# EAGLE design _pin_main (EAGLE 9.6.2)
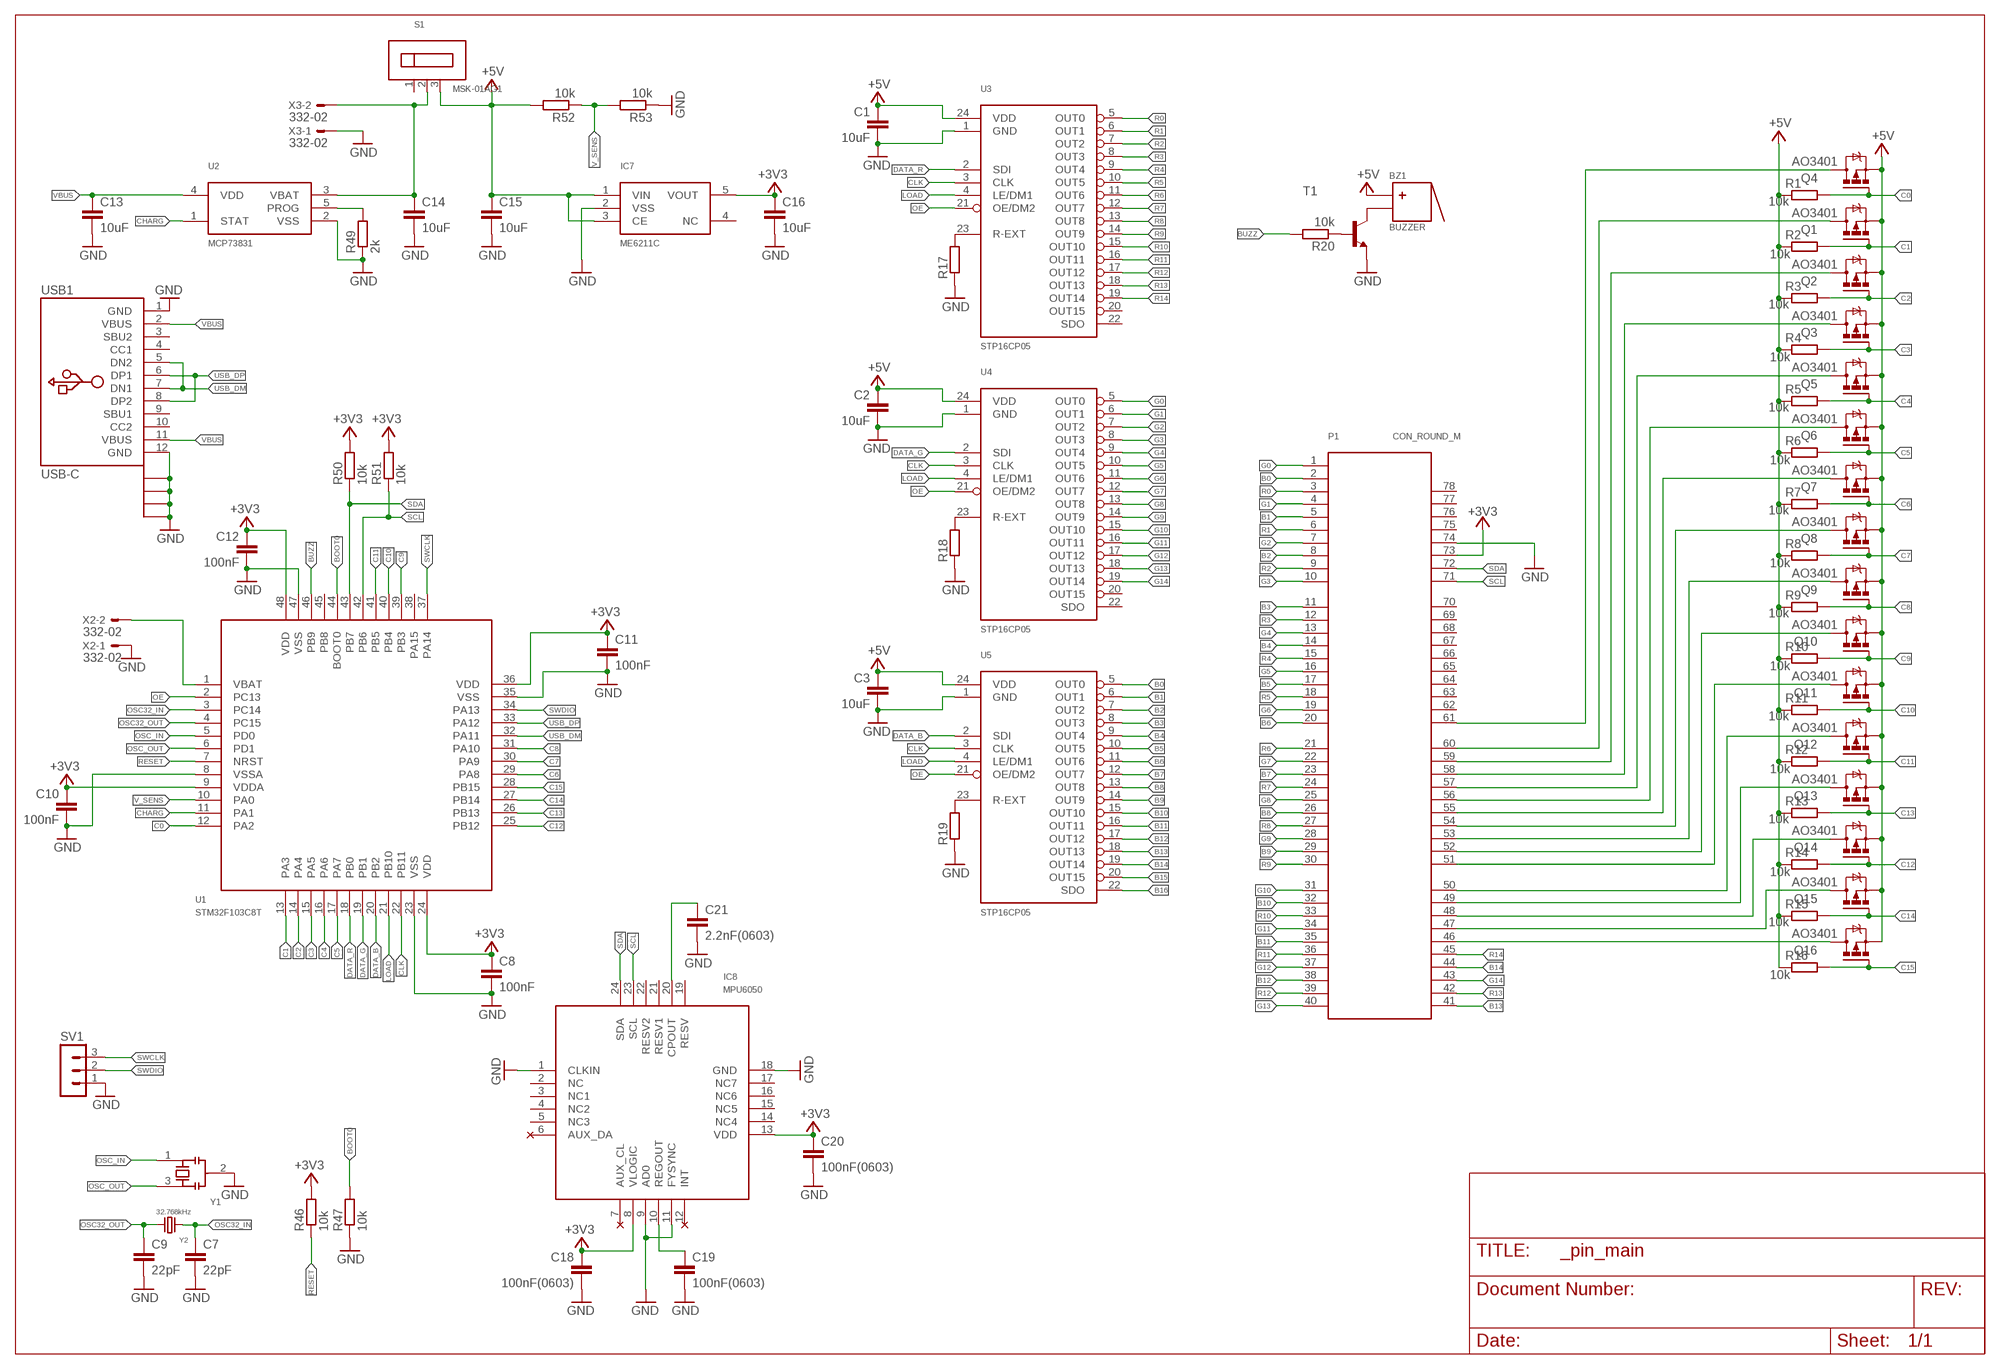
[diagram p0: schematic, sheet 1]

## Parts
BZ1  BUZZER  [HCT9032B]
C1  10uF  C-EUC0402K  [C0402K]
C2  10uF  C-EUC0402K  [C0402K]
C3  10uF  C-EUC0402K  [C0402K]
C7  22pF  C-EUC0402K  [C0402K]
C8  100nF  C-EUC0402K  [C0402K]
C9  22pF  C-EUC0402K  [C0402K]
C10  100nF  C-EUC0402K  [C0402K]
C11  100nF  C-EUC0402K  [C0402K]
C12  100nF  C-EUC0402K  [C0402K]
C13  10uF  C-EUC0805  [C0805]
C14  10uF  C-EUC0805  [C0805]
C15  10uF  C-EUC0805  [C0805]
C16  10uF  C-EUC0805  [C0805]
C18  100nF(0603)  C-EUC0402K  [C0402K]
C19  100nF(0603)  C-EUC0402K  [C0402K]
C20  100nF(0603)  C-EUC0402K  [C0402K]
C21  2.2nF(0603)  C-EUC0402K  [C0402K]
IC7  ME6211C  [SOT23-5]
IC8  MPU6050  [QFN24-4X4]
P1  CON_ROUND_M  [CON_61_M]
Q1  AO3401  IRLML5203  [MICRO3]
Q2  AO3401  IRLML5203  [MICRO3]
Q3  AO3401  IRLML5203  [MICRO3]
Q4  AO3401  IRLML5203  [MICRO3]
Q5  AO3401  IRLML5203  [MICRO3]
Q6  AO3401  IRLML5203  [MICRO3]
Q7  AO3401  IRLML5203  [MICRO3]
Q8  AO3401  IRLML5203  [MICRO3]
Q9  AO3401  IRLML5203  [MICRO3]
Q10  AO3401  IRLML5203  [MICRO3]
Q11  AO3401  IRLML5203  [MICRO3]
Q12  AO3401  IRLML5203  [MICRO3]
Q13  AO3401  IRLML5203  [MICRO3]
Q14  AO3401  IRLML5203  [MICRO3]
Q15  AO3401  IRLML5203  [MICRO3]
Q16  AO3401  IRLML5203  [MICRO3]
R1  10k  R-EU_R0402  [R0402]
R2  10k  R-EU_R0402  [R0402]
R3  10k  R-EU_R0402  [R0402]
R4  10k  R-EU_R0402  [R0402]
R5  10k  R-EU_R0402  [R0402]
R6  10k  R-EU_R0402  [R0402]
R7  10k  R-EU_R0402  [R0402]
R8  10k  R-EU_R0402  [R0402]
R9  10k  R-EU_R0402  [R0402]
R10  10k  R-EU_R0402  [R0402]
R11  10k  R-EU_R0402  [R0402]
R12  10k  R-EU_R0402  [R0402]
R13  10k  R-EU_R0402  [R0402]
R14  10k  R-EU_R0402  [R0402]
R15  10k  R-EU_R0402  [R0402]
R16  10k  R-EU_R0402  [R0402]
R17  R-EU_R0603  [R0603]
R18  R-EU_R0603  [R0603]
R19  R-EU_R0603  [R0603]
R20  10k  R-EU_R0402  [R0402]
R46  10k  R-EU_R0402  [R0402]
R47  10k  R-EU_R0402  [R0402]
R49  2k  R-EU_R0603  [R0603]
R50  10k  R-EU_R0402  [R0402]
R51  10k  R-EU_R0402  [R0402]
R52  10k  R-EU_R0402  [R0402]
R53  10k  R-EU_R0402  [R0402]
S1  MSK-01AG1  [MSK-01AG1]
SV1  MA03-1  [MA03-1]
T1  BC849-NPN-SOT23-BEC  [SOT23-BEC]
U1  STM32F103C8T  [LQFP48-7X7]
U2  MCP73831  [SOT23-5]
U3  STP16CP05  [TSSOP24]
U4  STP16CP05  [TSSOP24]
U5  STP16CP05  [TSSOP24]
USB1  USB-C  [USB-C-A40-00119]
X2  332-02  [332-02]
X3  332-02  [332-02]
Y1  XTAL_CSTCE  [CSTCE]
Y2  32.768kHz  WE-XTAL_WATCH_830002997B_2X6  [WE-XTAL_WATCH-2X6]

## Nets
+3V3: C8.1 C10.1 C11.1 C12.1 C16.1 C18.1 C20.1 IC7.5(VOUT) IC8.8(VLOGIC) IC8.13(VDD) P1.73 R46.2 R50.2 R51.2 U1.9(VDDA) U1.24(VDD) U1.36(VDD) U1.48(VDD)
+5V: BZ1.1 C1.1 C2.1 C3.1 C15.1 IC7.1(VIN) IC7.3(CE) Q1.2(S) Q2.2(S) Q3.2(S) Q4.2(S) Q5.2(S) Q6.2(S) Q7.2(S) Q8.2(S) Q9.2(S) Q10.2(S) Q11.2(S) Q12.2(S) Q13.2(S) Q14.2(S) Q15.2(S) Q16.2(S) R1.1 R2.1 R3.1 R4.1 R5.1 R6.1 R7.1 R8.1 R9.1 R10.1 R11.1 R12.1 R13.1 R14.1 R15.1 R16.1 R52.2 S1.3 U3.24(VDD) U4.24(VDD) U5.24(VDD)
B0: P1.2 U5.5(OUT0)
B1: P1.5 U5.6(OUT1)
B2: P1.8 U5.7(OUT2)
B3: P1.11 U5.8(OUT3)
B4: P1.14 U5.9(OUT4)
B5: P1.17 U5.10(OUT5)
B6: P1.20 U5.11(OUT6)
B7: P1.23 U5.12(OUT7)
B8: P1.26 U5.13(OUT8)
B9: P1.29 U5.14(OUT9)
B10: P1.32 U5.15(OUT10)
B11: P1.35 U5.16(OUT11)
B12: P1.38 U5.17(OUT12)
B13: P1.41 U5.18(OUT13)
B14: P1.44 U5.19(OUT14)
B15: U5.20(OUT15)
B16: U5.22(SDO)
BOOT0: R47.2 U1.44(BOOT0)
BUZZ: R20.2 U1.46(PB9)
C0: Q4.1(G) R1.2 U1.12(PA2)
C1: Q1.1(G) R2.2 U1.13(PA3)
C2: Q2.1(G) R3.2 U1.14(PA4)
C3: Q3.1(G) R4.2 U1.15(PA5)
C4: Q5.1(G) R5.2 U1.16(PA6)
C5: Q6.1(G) R6.2 U1.17(PA7)
C6: Q7.1(G) R7.2 U1.29(PA8)
C7: Q8.1(G) R8.2 U1.30(PA9)
C8: Q9.1(G) R9.2 U1.31(PA10)
C9: Q10.1(G) R10.2 U1.39(PB3)
C10: Q11.1(G) R11.2 U1.40(PB4)
C11: Q12.1(G) R12.2 U1.41(PB5)
C12: Q14.1(G) R14.2 U1.25(PB12)
C13: Q13.1(G) R13.2 U1.26(PB13)
C14: Q15.1(G) R15.2 U1.27(PB14)
C15: Q16.1(G) R16.2 U1.28(PB15)
CHARG: U1.11(PA1) U2.1(STAT)
CLK: U1.22(PB11) U3.3(CLK) U4.3(CLK) U5.3(CLK)
DATA_B: U1.20(PB2) U5.2(SDI)
DATA_G: U1.19(PB1) U4.2(SDI)
DATA_R: U1.18(PB0) U3.2(SDI)
G0: P1.1 U4.5(OUT0)
G1: P1.4 U4.6(OUT1)
G2: P1.7 U4.7(OUT2)
G3: P1.10 U4.8(OUT3)
G4: P1.13 U4.9(OUT4)
G5: P1.16 U4.10(OUT5)
G6: P1.19 U4.11(OUT6)
G7: P1.22 U4.12(OUT7)
G8: P1.25 U4.13(OUT8)
G9: P1.28 U4.14(OUT9)
G10: P1.31 U4.15(OUT10)
G11: P1.34 U4.16(OUT11)
G12: P1.37 U4.17(OUT12)
G13: P1.40 U4.18(OUT13)
G14: P1.43 U4.19(OUT14)
GND: C1.2 C2.2 C3.2 C7.2 C8.2 C9.2 C10.2 C11.2 C12.2 C13.2 C14.2 C15.2 C16.2 C18.2 C19.2 C20.2 C21.2 IC7.2(VSS) IC8.1(CLKIN) IC8.9(AD0) IC8.11(FYSYNC) IC8.18(GND) P1.74 R17.1 R18.1 R19.1 R47.1 R49.1 R53.1 SV1.1 T1.E U1.8(VSSA) U1.23(VSS) U1.35(VSS) U1.47(VSS) U2.2(VSS) U3.1(GND) U4.1(GND) U5.1(GND) USB1.1(GND) USB1.12(GND) USB1.A(EXT) USB1.B(EXT1) USB1.C(EXT2) USB1.D(EXT3) X2.1 X3.1 Y1.2(GND)
LOAD: U1.21(PB10) U3.4(LE/DM1) U4.4(LE/DM1) U5.4(LE/DM1)
N$1: R17.2 U3.23(R-EXT)
N$2: R18.2 U4.23(R-EXT)
N$3: R19.2 U5.23(R-EXT)
N$4: BZ1.2 T1.C
N$5: R20.1 T1.B
N$49: U1.1(VBAT) X2.2
N$50: P1.46 Q16.3(D)
N$51: R49.2 U2.5(PROG)
N$52: C19.1 IC8.10(REGOUT)
N$53: C21.1 IC8.20(CPOUT)
N$54: P1.47 Q15.3(D)
N$55: C14.1 S1.2 U2.3(VBAT) X3.2
N$56: P1.48 Q14.3(D)
N$57: P1.49 Q13.3(D)
N$58: P1.50 Q12.3(D)
N$59: P1.51 Q11.3(D)
N$60: P1.52 Q10.3(D)
N$61: P1.53 Q9.3(D)
N$62: P1.54 Q8.3(D)
N$63: P1.55 Q7.3(D)
N$64: P1.56 Q6.3(D)
N$65: P1.57 Q5.3(D)
N$66: P1.58 Q3.3(D)
N$67: P1.59 Q2.3(D)
N$68: P1.60 Q1.3(D)
N$69: P1.61 Q4.3(D)
OE: U1.2(PC13) U3.21(OE/DM2) U4.21(OE/DM2) U5.21(OE/DM2)
OSC32_IN: C7.1 U1.3(PC14) Y2.1
OSC32_OUT: C9.1 U1.4(PC15) Y2.2
OSC_IN: U1.5(PD0) Y1.1(XI)
OSC_OUT: U1.6(PD1) Y1.3(XO)
R0: P1.3 U3.5(OUT0)
R1: P1.6 U3.6(OUT1)
R2: P1.9 U3.7(OUT2)
R3: P1.12 U3.8(OUT3)
R4: P1.15 U3.9(OUT4)
R5: P1.18 U3.10(OUT5)
R6: P1.21 U3.11(OUT6)
R7: P1.24 U3.12(OUT7)
R8: P1.27 U3.13(OUT8)
R9: P1.30 U3.14(OUT9)
R10: P1.33 U3.15(OUT10)
R11: P1.36 U3.16(OUT11)
R12: P1.39 U3.17(OUT12)
R13: P1.42 U3.18(OUT13)
R14: P1.45 U3.19(OUT14)
RESET: R46.1 U1.7(NRST)
SCL: IC8.23(SCL) P1.71 R51.1 U1.42(PB6)
SDA: IC8.24(SDA) P1.72 R50.1 U1.43(PB7)
SWCLK: SV1.3 U1.37(PA14)
SWDIO: SV1.2 U1.34(PA13)
USB_DM: U1.32(PA11) USB1.5(DN2) USB1.7(DN1)
USB_DP: U1.33(PA12) USB1.6(DP1) USB1.8(DP2)
V_SENS: R52.1 R53.2 U1.10(PA0)
VBUS: C13.1 U2.4(VDD) USB1.2(VBUS) USB1.11(VBUS)
Unconnected: IC7.4(NC) IC8.2(NC) IC8.3(NC1) IC8.4(NC2) IC8.5(NC3) IC8.6(AUX_DA) IC8.7(AUX_CL) IC8.12(INT) IC8.14(NC4) IC8.15(NC5) IC8.16(NC6) IC8.17(NC7) IC8.19(RESV) IC8.21(RESV1) IC8.22(RESV2) P1.62 P1.63 P1.64 P1.65 P1.66 P1.67 P1.68 P1.69 P1.70 P1.75 P1.76 P1.77 P1.78 S1.1 U1.38(PA15) U1.45(PB8) U3.20(OUT15) U3.22(SDO) U4.20(OUT15) U4.22(SDO) USB1.3(SBU2) USB1.4(CC1) USB1.9(SBU1) USB1.10(CC2)

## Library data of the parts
BZ1 = GUIDO_PCB_LIB:BUZZER
C1-C3 C7-C16 C18-C21 = my_rcl:C-EU: CAPACITOR, European symbol; SPICEPREFIX: C
IC7 = GUIDO_PCB_LIB:ME6211C
IC8 = controller_KRAI:MPU6050
P1 = GUIDO_PCB_LIB:CON_ROUND_M
Q1-Q16 = transistor-power:IRLML5203: HEXFET P-Channel Power MOSFET
R1-R20 R46 R47 R49-R53 = my_rcl:R-EU_: RESISTOR, European symbol; SPICEPREFIX: R
S1 = GUIDO_PCB_LIB:MSK-01AG1
SV1 = my_con-lstb:MA03-1: PIN HEADER; OC_FARNELL: unknown; OC_NEWARK: unknown
T1 = transistor-neu-to92:*-NPN-: NPN Transistror
U1 = GUIDO_PCB_LIB:STM32F103C8T
U2 = GUIDO_PCB_LIB:MCP73831
U3-U5 = GUIDO_PCB_LIB:STP16CP05
USB1 = GUIDO_PCB_LIB:USB-C
X2 X3 = con-garry:332-02: 2 Pin - 2mm Dual Row
Y1 = GUIDO_PCB_LIB:XTAL_CSTCE
Y2 = my_Wurth_Quartz Crystals & Oscillators_WE-XTAL:WE-XTAL_WATCH: WE-XTAL Watch Crystals; C-LOAD: 12.5pF; DATASHEET-URL: https://www.we-online.com/catalog/datasheet/830002997B.pdf; MOUNT: THT; PART-NUMBER: 830002997B; TOLERANCE: ±20ppm

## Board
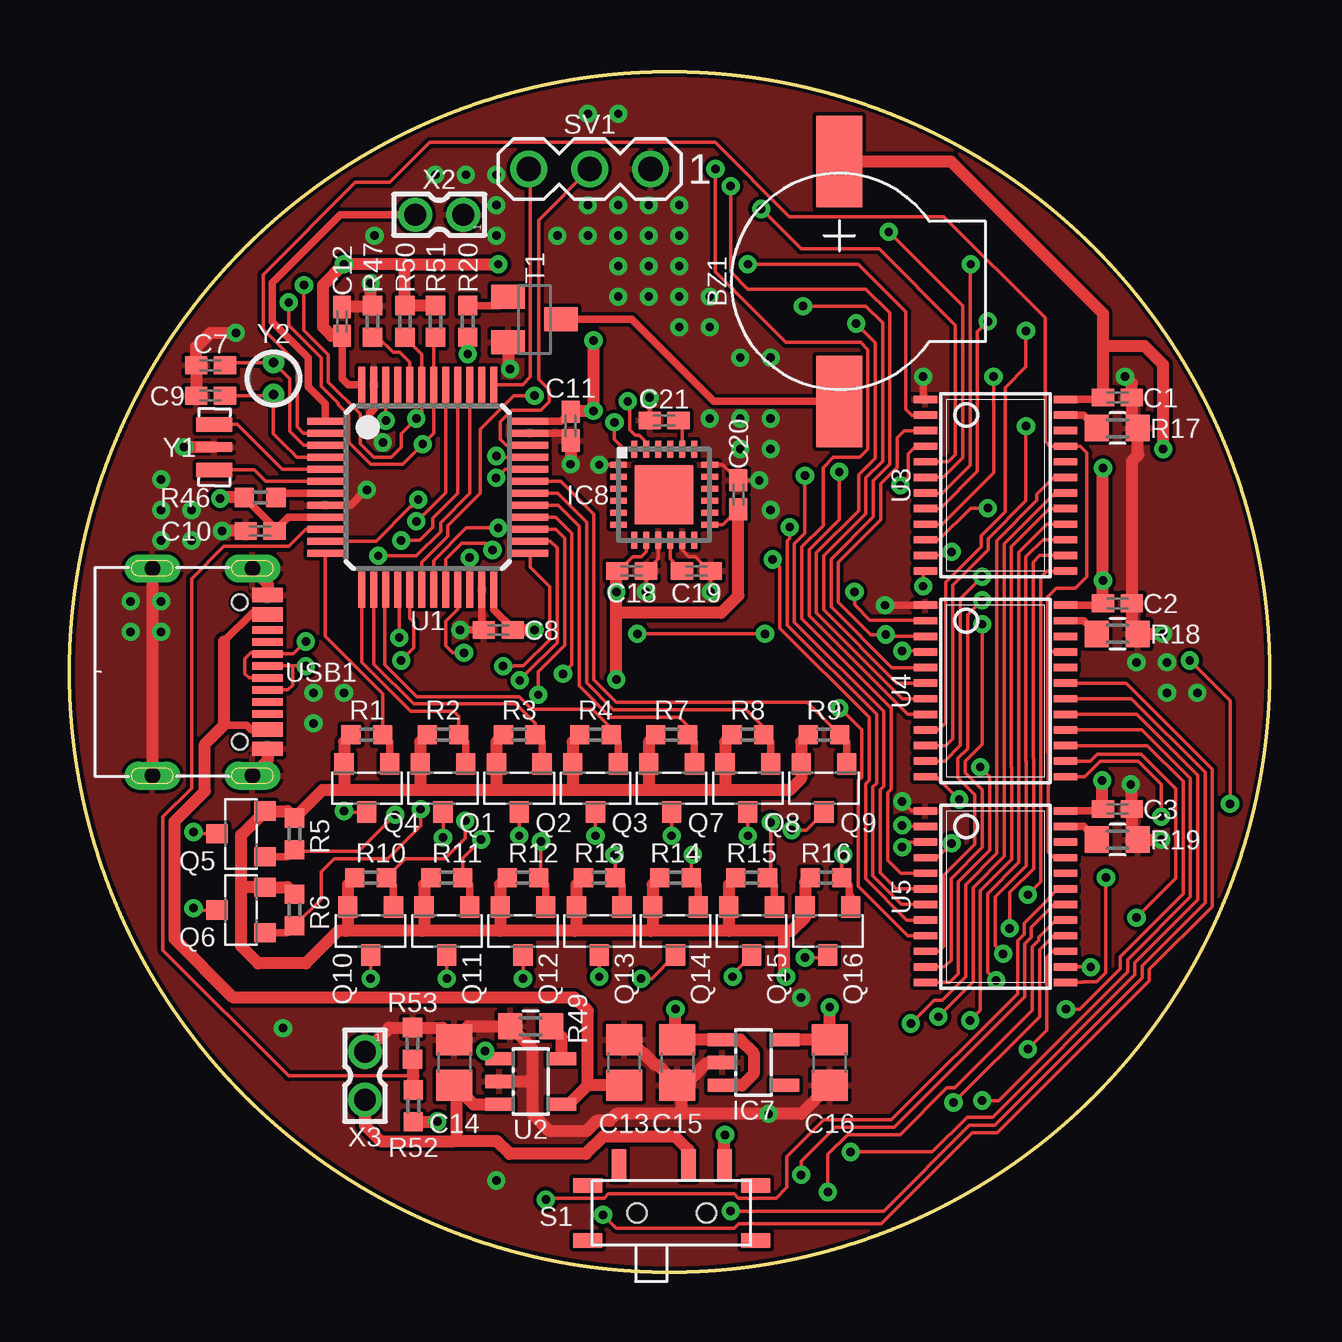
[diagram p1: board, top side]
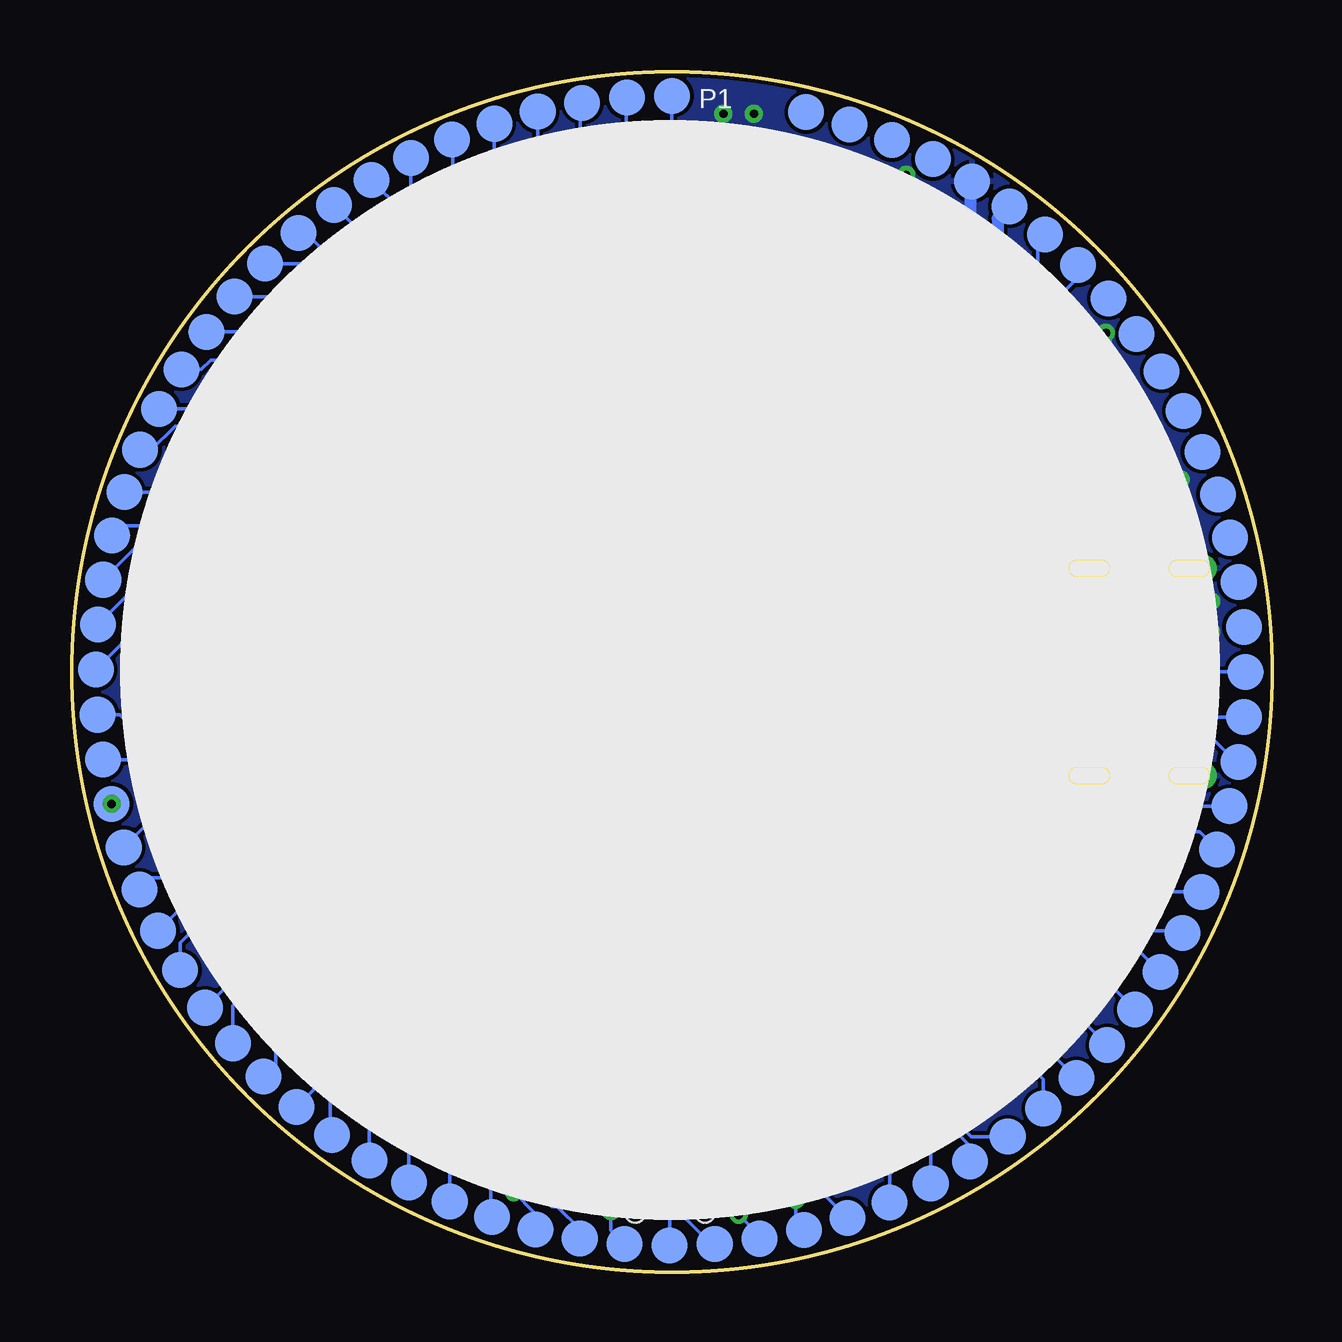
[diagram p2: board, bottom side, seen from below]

Size 50 x 50 mm. Coordinates in mm from the lower left corner, seen from the top.
Outline: circle at 25,25 radius 25
Copper layers (1*16): Top 0.035mm / dielectric 0.8mm / Bottom 0.035mm
Design rules "default *": minimum track width 6mil, minimum drill 0.35mm, track to track 6mil, track to pad 6mil, pad to pad 6mil, via to via 6mil, smd to smd 6mil, copper to edge 6mil, drill to drill 6mil, minimum pad ring 10mil, minimum via ring 8mil, stop-mask expansion 4mil, vias tented up to drill 0.35mm, thermal gap 6mil

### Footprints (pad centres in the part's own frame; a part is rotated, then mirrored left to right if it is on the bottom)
HCT9032B = smd 1.93 x 3.81: 1 0,5; 2 0,-5
C0402K = smd 0.925 x 0.74: 1 -0.6,0; 2 0.6,0
C0805 = smd 1.3 x 1.5: 1 -0.95,0; 2 0.95,0
SOT23-5 = smd 0.55 x 1.2: 1 -0.95,-1.3; 2 0,-1.3; 3 0.95,-1.3; 4 0.95,1.3; 5 -0.95,1.3
QFN24-4X4 = smd 0.7 x 0.25: 1 -1.9,1.25; 2 -1.9,0.75; 3 -1.9,0.25; 4 -1.9,-0.25; 5 -1.9,-0.75; 6 -1.9,-1.25; 13 1.9,-1.25; 14 1.9,-0.75; 15 1.9,-0.25; 16 1.9,0.25; 17 1.9,0.75; 18 1.9,1.25 | smd 0.25 x 0.7: 7 -1.25,-1.9; 8 -0.75,-1.9; 9 -0.25,-1.9; 10 0.25,-1.9; 11 0.75,-1.9; 12 1.25,-1.9; 19 1.25,1.9; 20 0.75,1.9; 21 0.25,1.9; 22 -0.25,1.9; 23 -0.75,1.9; 24 -1.25,1.9 | smd 2.45 x 2.45: EXP 0,0
CON_61_M = smd 1.5 x 1.5 bottom: 1 -24,0; 2 -23.93,1.879; 3 -23.713,3.747; 4 -23.35,5.593; 5 -22.843,7.404; 6 -22.195,9.17; 7 -21.412,10.879; 8 -20.496,12.522; 9 -19.454,14.088; 10 -18.293,15.567; 11 -17.019,16.95; 12 -15.641,18.23; 13 -14.166,19.397; 14 -12.605,20.445; 15 -10.966,21.367; 16 -9.259,22.158; 17 -7.496,22.813; 18 -5.687,23.327; 19 -3.843,23.698; 20 -1.976,23.922; 21 -0.097,24; 22 1.782,23.93; 23 3.65,23.713; 24 5.495,23.35; 25 7.307,22.843; 26 9.072,22.195; 27 10.782,21.412; 28 12.425,20.496; 29 13.99,19.454; 30 15.47,18.293; 31 16.853,17.019; 32 18.133,15.641; 33 19.3,14.166; 34 20.348,12.605; 35 21.27,10.966; 36 22.061,9.259; 37 22.716,7.496; 38 23.23,5.687; 39 23.6,3.844; 40 23.825,1.976; 41 23.903,0.097; 42 23.833,-1.782; 43 23.616,-3.65; 44 23.252,-5.495; 45 22.746,-7.306; 46 22.098,-9.072; 47 21.314,-10.782; 48 20.399,-12.424; 49 19.357,-13.99; 50 18.196,-15.47; 51 16.922,-16.853; 52 15.544,-18.133; 53 14.069,-19.3; 54 12.507,-20.348; 55 10.868,-21.27; 56 9.162,-22.061; 57 7.399,-22.715; 58 5.59,-23.23; 59 3.746,-23.6; 60 1.879,-23.825; 61 0,-23.903; 62 -1.879,-23.833; 63 -3.747,-23.615; 64 -5.593,-23.252; 65 -7.404,-22.746; 66 -9.169,-22.098; 67 -10.879,-21.314; 68 -12.522,-20.399; 69 -14.088,-19.357; 70 -15.567,-18.196; 71 -16.95,-16.922; 72 -18.23,-15.544; 73 -19.397,-14.069; 74 -20.445,-12.507; 75 -21.367,-10.868; 76 -22.158,-9.162; 77 -22.813,-7.399; 78 -23.327,-5.59
MICRO3 = smd 0.8 x 0.9: 1 -0.95,-1; 2 0.95,-1; 3 0,1
R0402 = smd 0.8 x 0.8: 1 -0.659,0; 2 0.659,0
R0603 = smd 1 x 1.1: 1 -0.85,0; 2 0.85,0
MSK-01AG1 = smd 1.3 x 0.6: 1 2,2.2; 2 2,-0.7; 3 2,-2.2 | smd 0.6 x 1.2: 4 1.15,3.5; 5 -1.15,3.5; 6 -1.15,-3.5; 7 1.15,-3.5 | hole 0.8: 0,1.45; 0,-1.45
MA03-1 = drill 1.016: 1 -2.54,0; 2 0,0; 3 2.54,0
SOT23-BEC = smd 1 x 1.4: B -0.95,-1.1; C 0,1.1; E 0.95,-1.1
LQFP48-7X7 = smd 1.5 x 0.3: 1 -4.268,2.75; 2 -4.268,2.25; 3 -4.268,1.75; 4 -4.268,1.25; 5 -4.268,0.75; 6 -4.268,0.25; 7 -4.268,-0.25; 8 -4.268,-0.75; 9 -4.268,-1.25; 10 -4.268,-1.75; 11 -4.268,-2.25; 12 -4.268,-2.75; 25 4.268,-2.75; 26 4.268,-2.25; 27 4.268,-1.75; 28 4.268,-1.25; 29 4.268,-0.75; 30 4.268,-0.25; 31 4.268,0.25; 32 4.268,0.75; 33 4.268,1.25; 34 4.268,1.75; 35 4.268,2.25; 36 4.268,2.75 | smd 0.3 x 1.5: 13 -2.75,-4.268; 14 -2.25,-4.268; 15 -1.75,-4.268; 16 -1.25,-4.268; 17 -0.75,-4.268; 18 -0.25,-4.268; 19 0.25,-4.268; 20 0.75,-4.268; 21 1.25,-4.268; 22 1.75,-4.268; 23 2.25,-4.268; 24 2.75,-4.268; 37 2.75,4.268; 38 2.25,4.268; 39 1.75,4.268; 40 1.25,4.268; 41 0.75,4.268; 42 0.25,4.268; 43 -0.25,4.268; 44 -0.75,4.268; 45 -1.25,4.268; 46 -1.75,4.268; 47 -2.25,4.268; 48 -2.75,4.268
TSSOP24 = smd 0.305 x 0.991: 1 -3.575,-2.918; 2 -2.925,-2.918; 3 -2.275,-2.918; 4 -1.625,-2.918; 5 -0.975,-2.918; 6 -0.325,-2.918; 7 0.325,-2.918; 8 0.975,-2.918; 9 1.625,-2.918; 10 2.275,-2.918; 11 2.925,-2.918; 12 3.575,-2.918; 13 3.575,2.918; 14 2.925,2.918; 15 2.275,2.918; 16 1.625,2.918; 17 0.975,2.918; 18 0.325,2.918; 19 -0.325,2.918; 20 -0.975,2.918; 21 -1.625,2.918; 22 -2.275,2.918; 23 -2.925,2.918; 24 -3.575,2.918
USB-C-A40-00119 = smd 0.6 x 1.27: 1 -3.2,7.2; 2 -2.4,7.2; 11 2.4,7.2; 12 3.2,7.2 | smd 0.3 x 1.27: 3 -1.75,7.2; 4 -1.25,7.2; 5 -0.75,7.2; 6 -0.25,7.2; 7 0.25,7.2; 8 0.75,7.2; 9 1.25,7.2; 10 1.75,7.2 | drill 0.65 pad 1 long: A -4.32,6.57; B -4.32,2.4; C 4.32,2.4; D 4.32,6.57 | hole 0.65: -2.9,6.05; 2.9,6.05
332-02 = drill 0.9 pad 1.27: 1 0,-1; 2 0,1
CSTCE = smd 0.6 x 1.5: 1 -0.95,0; 3 0.95,0 | smd 0.4 x 1.5: 2 0,0
WE-XTAL_WATCH-2X6 = drill 0.4 pad 0.6: 1 -0.667,0; 2 0.667,0

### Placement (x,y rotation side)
BZ1  32.07,41.27 0 top
C1  43.66,36.43 0 top
C2  43.66,27.86 0 top
C3  43.66,19.29 0 top
C7  5.87,37.78 180 top
C8  17.86,26.75 180 top
C9  5.87,36.51 180 top
C10  7.94,30.88 180 top
C11  20.88,35.24 270 top
C12  11.35,39.61 90 top
C13  23.1,8.73 90 top
C14  16.03,8.73 90 top
C15  25.32,8.73 270 top
C16  31.67,8.73 270 top
C18  23.42,29.21 0 top
C19  26.11,29.21 0 top
C20  27.86,32.38 90 top
C21  24.77,35.48 180 top
IC7  28.5,8.73 270 top
IC8  24.77,32.38 0 top
P1  25,25 270 top
Q1  15.56,20.16 180 top
Q2  18.73,20.16 180 top
Q3  21.91,20.16 180 top
Q4  12.38,20.16 180 top
Q5  7.14,18.26 90 top
Q6  7.14,15.08 90 top
Q7  25.08,20.16 180 top
Q8  28.26,20.16 180 top
Q9  31.43,20.16 180 top
Q10  12.54,14.21 180 top
Q11  15.72,14.21 180 top
Q12  18.89,14.21 180 top
Q13  22.07,14.21 180 top
Q14  25.24,14.21 180 top
Q15  28.42,14.21 180 top
Q16  31.59,14.21 180 top
R1  12.38,22.38 0 top
R2  15.56,22.38 0 top
R3  18.73,22.38 0 top
R4  21.91,22.38 0 top
R5  9.37,18.26 270 top
R6  9.37,15.08 270 top
R7  25.08,22.38 0 top
R8  28.26,22.38 0 top
R9  31.43,22.38 0 top
R10  12.54,16.43 0 top
R11  15.72,16.43 0 top
R12  18.89,16.43 0 top
R13  22.07,16.43 0 top
R14  25.24,16.43 0 top
R15  28.42,16.43 0 top
R16  31.51,16.43 0 top
R17  43.66,35.16 180 top
R18  43.66,26.59 180 top
R19  43.66,18.02 180 top
R20  16.59,39.61 270 top
R46  7.94,32.27 180 top
R47  12.62,39.61 270 top
R49  19.21,10.24 0 top
R50  13.97,39.61 90 top
R51  15.24,39.61 90 top
R52  14.32,6.92 270 top
R53  14.29,9.53 270 top
S1  25.08,2.46 90 top
SV1  21.67,45.96 180 top
T1  19.37,39.69 270 top
U1  14.92,32.7 0 top
U2  19.21,7.94 270 top
U3  38.58,32.78 270 top
U4  38.58,24.21 270 top
U5  38.58,15.64 270 top
USB1  1.05,25 270 top
X2  15.4,44.05 90 top
X3  12.3,8.18 180 top
Y1  6.03,34.37 270 top
Y2  8.49,37.23 270 top

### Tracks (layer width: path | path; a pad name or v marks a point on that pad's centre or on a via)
+3V3  (via drill 0.35)
  Top 0.152: C20.1 27.21,31.14 IC8.13 | IC8.8 24.02,30.01 23.81,29.81 23.46,29.81 22.82,29.18 22.78,29.18
  Top 0.305: U1.36 20.49,35.45 C11.1 | U1.24 17.67,27.6 18.46,26.81 C8.1 | U1.9 9.11,31.45 C10.1 8.54,31.02 R46.2 | C12.1 11.35,37.23 11.61,36.97 U1.48
  Top 0.508: R51.2 R50.2 13.97,41.98 | C11.1 20.91,35.88 v21.83,35.88 v21.83,38.81 | C18.1 22.78,29.18 v22.78,28.34 22.78,27.54 | C20.1 27.86,28.18 27.15,27.46 22.86,27.46 22.78,27.54 | IC7.5 C16.1 v31.67,11.03 | v22.78,24.69 22.78,27.54 | R46.2 6.32,32.27 v6.27,32.23 | C12.1 10.92,39.01 10.56,39.37 10.56,41.12 v11.43,41.99 v11.44,41.98 13.97,41.98 | 13.97,41.98 13.98,41.99 v17.86,41.99 | C8.1 v19.37,26.75
  Bottom 0.508: v31.67,11.03 33.18,12.54 33.18,17.67 26.16,24.69 v22.78,24.69 22.07,24.69 20,26.75 v19.37,26.75 | P1.73 11.43,43.9 v11.43,41.99 11.47,41.95 11.47,34.41 9.29,32.23 v6.27,32.23 | v17.86,41.99 20.8,41.99 21.83,40.96 v21.83,38.81 | v22.78,28.34 21.2,28.34 19.61,29.94 19.61,33.66 v21.83,35.88
+5V  (via drill 0.35)
  Top 0.305: U3.24 42.98,36.36 C1.1 | U4.24 42.98,27.78 C2.1 | U5.24 42.98,19.21 C3.1
  Top 0.508: R6.1 9.07,16.03 Q6.2 7.15,16.03 7.14,16.03 | R10.1 11.59,16.14 Q10.2 11.59,14.29 11.51,14.21 | R11.1 14.77,16.14 Q11.2 14.77,14.29 14.68,14.21 | R12.1 17.94,16.14 Q12.2 17.94,14.21 | R13.1 21.12,16.14 Q13.2 21.12,14.29 21.03,14.21 | R14.1 24.29,16.14 Q14.2 24.29,14.29 24.21,14.21 | R15.1 27.47,16.14 Q15.2 27.47,14.21 27.46,14.21 | R16.1 30.64,16.22 Q16.2 30.64,14.77 30.08,14.21 29.77,14.21 | R9.1 30.48,22.09 Q9.2 30.48,20.56 30,20.08 27.3,20.08 | R8.1 27.31,22.09 Q8.2 27.31,20.08 27.3,20.08 | R7.1 24.13,22.09 Q7.2 24.13,20.08 | R4.1 20.96,22.09 Q3.2 20.96,20.08 20.95,20.08 | R3.1 17.78,22.09 Q2.2 17.78,20.16 17.7,20.08 | R2.1 14.61,22.09 Q1.2 14.61,20.16 14.53,20.08 | R1.1 11.43,22.09 Q4.2 11.43,20.16 11.35,20.08 | 29.77,14.21 27.46,14.21 | 27.46,14.21 24.21,14.21 | 24.21,14.21 21.03,14.21 | 21.03,14.21 17.94,14.21 | 17.94,14.21 14.68,14.21 | 14.68,14.21 11.51,14.21 | 11.51,14.21 11.19,14.21 9.84,12.86 7.86,12.86 7.14,13.57 7.14,16.03 | 7.14,16.03 7.14,18.21 Q5.2 9.07,19.21 R5.1 10.53,20.08 11.35,20.08 | 27.3,20.08 24.13,20.08 | 24.13,20.08 20.95,20.08 | 20.95,20.08 17.7,20.08 | 17.7,20.08 14.53,20.08 | 14.53,20.08 11.35,20.08 | 43.06,38.58 C1.1 | C2.1 v43.06,28.81 v43.06,33.5 | 43.06,38.58 44.79,38.58 45.56,37.8 v45.56,34.29 | C3.1 43.02,19.32 v43.02,20.48 | IC7.3 28.02,7.78 28.5,8.26 28.5,9.13 27.94,9.68 IC7.1 C15.1 25.24,9.76 v25.24,10.95 | S1.3 27.28,5.69 v27.3,5.71 | v29.84,12.3 29.77,12.38 29.77,14.21 | R52.2 v15.31,6.26 v15.32,6.27 | BZ1.1 36.72,46.27 43.06,39.94 43.06,38.58
  Bottom 0.508: v43.02,20.48 43.02,23.02 | 43.02,23.02 43.02,28.78 v43.06,28.81 | v45.56,34.29 45.56,34.37 44.69,33.5 v43.06,33.5 | 27.38,10.95 28.73,10.95 29.84,12.06 v29.84,12.3 | v27.3,5.71 27.3,6.27 | 27.3,6.27 27.3,7.46 | 27.3,7.46 27.3,10.87 27.38,10.95 | v25.24,10.95 27.38,10.95 | v15.32,6.27 27.3,6.27 | 43.02,23.02 37.39,23.02 36.12,21.75 36.12,19.45 36.66,18.9 37.14,18.9 37.62,18.41 37.62,15.48 29.61,7.46 27.3,7.46
B0  (via drill 0.35)
  Top 0.152: U5.5 34.63,16.61 34.08,17.16 34.08,19.96 34.23,20.11 34.23,23.48 30.51,27.21 30.51,30.21 31.39,31.1 31.39,33.52 31.82,33.94 32.93,33.94 33.26,34.27 33.26,38.43 32.96,38.73 29.84,38.73 26.91,41.67 v26.91,45.96
  Bottom 0.152: P1.2 26.91,48.9 v26.91,45.96
B1  (via drill 0.35)
  Top 0.152: U5.6 34.44,15.96 33.77,16.63 33.77,20.09 33.92,20.24 33.92,23.36 30.2,27.08 30.2,30.34 30.64,30.77 v30.64,33.18
  Bottom 0.152: P1.5 32.4,40.4 30.64,38.64 v30.64,33.18
B2  (via drill 0.35)
  Top 0.152: U5.7 34.66,15.31 33.47,16.5 33.47,20.21 33.62,20.36 33.62,23.23 29.9,26.96 29.9,30.46 30,30.57 v30,31.04
  Bottom 0.152: v30,31.04 31.46,32.49 31.46,35.36 36.23,40.13 36.23,44.21 P1.8
B3  (via drill 0.35)
  Top 0.152: U5.8 34.88,14.66 33.17,16.38 33.17,20.34 33.32,20.49 33.32,23.11 29.59,26.83 29.59,29.38 v29.29,29.69
  Bottom 0.152: P1.11 39.81,42.02 38.74,40.95 37.91,40.95 32.88,35.91 32.88,32.57 29.99,29.69 v29.29,29.69
B4  (via drill 0.35)
  Top 0.152: U5.9 34.91,14.01 32.86,16.06 32.86,20.47 33.01,20.62 33.01,22.59 32.1,23.5 v32.07,23.5
  Bottom 0.152: P1.14 44.61,37.6 44.23,37.99 41.87,37.99 41.7,37.83 39.99,37.83 39.23,38.59 35.99,38.59 33.18,35.79 33.18,32.1 33.37,31.91 33.37,28.11 32.07,26.81 v32.07,23.5
B5  (via drill 0.35)
  Top 0.152: U5.10 36.22,13.36 36.42,13.56 36.42,16.52 37.72,17.82 37.72,19.89 37.01,20.6 37.01,21.41 37.41,21.81 37.41,27.38 v38.02,27.98
  Bottom 0.152: P1.17 37.97,32.5 37.41,31.94 37.41,28.59 v38.02,27.98
B6  (via drill 0.35)
  Top 0.152: U5.11 36.45,12.71 36.73,12.99 36.73,16.39 38.03,17.69 38.03,20.09 37.32,20.8 37.32,21.28 38.02,21.99 v38.02,26.99
  Bottom 0.152: P1.20 45.87,30.03 41.06,30.03 v38.02,26.99
B7  (via drill 0.35)
  Top 0.152: U5.12 36.67,12.06 37.03,12.43 37.03,16.27 38.33,17.57 38.33,20.64 v37.94,21.03
  Bottom 0.152: P1.23 46.57,21.35 44.63,19.41 39.57,19.41 v37.94,21.03
B8  (via drill 0.35)
  Top 0.152: U5.13 42.22,12.06 42.26,12.09 42.8,12.09 43.18,12.48 v43.18,16.43
  Bottom 0.152: v43.18,16.43 46.69,16.43 P1.26
B9  (via drill 0.35)
  Top 0.152: U5.14 42.53,12.71 v42.55,12.7
  Bottom 0.152: v42.55,12.7 42.76,12.7 P1.29
B10  (via drill 0.35)
  Top 0.152: U5.15 40.96,13.36 40.72,13.12 40.72,10.08 v39.93,9.29
  Bottom 0.152: v39.93,9.29 39.93,7.58 P1.32
B11  (via drill 0.35)
  Top 0.152: U5.16 41,14.01 40.69,13.7 40.69,13.69 40.41,13.42 40.41,10.63 36.84,7.06 v36.83,7.06
  Bottom 0.152: v36.83,7.06 35.97,6.2 P1.35
B12  (via drill 0.35)
  Top 0.152: U5.17 41.09,14.66 40.38,13.95 40.38,13.82 40.11,13.55 40.11,10.9 36.88,7.67 36.54,7.67 34.6,5.73 32.41,5.73 31.59,4.91 v31.59,3.33
  Bottom 0.152: v31.59,3.33 30.69,2.43 P1.38
B13  (via drill 0.35)
  Top 0.152: U5.18 41.03,15.31 40.08,14.36 40.08,13.94 39.8,13.67 39.8,11.47 34.37,6.03 31.91,6.03 30.48,4.6 v30.48,4.05
  Bottom 0.152: v30.48,4.05 29.61,3.17 25.96,3.17 25.1,2.32 P1.41
B14  (via drill 0.35)
  Top 0.152: U5.19 41.17,15.96 40.77,15.56 40.77,15.53 39.77,14.53 39.77,14.07 39.5,13.8 39.5,11.6 34.24,6.34 31.42,6.34 29.89,4.8 29.89,4.31 29.87,4.3 29.87,3.52 29.43,3.08 27.86,3.08 27.69,3.25 22.45,3.25 22.28,3.08 19.91,3.08 v19.84,3.02
  Bottom 0.152: v19.84,3.02 19.84,2.09 P1.44
BOOT0
  Top 0.152: U1.44 14.17,37.9 13.75,38.32 13.47,38.32 12.85,38.95 R47.2
BUZZ  (via drill 0.35)
  Top 0.152: R20.2 v16.59,38.25 | v13.18,35.48 v13.17,35.48 U1.46
  Bottom 0.152: v16.59,38.25 13.49,38.25 13.18,37.94 v13.18,35.48
C0
  Top 0.152: R1.2 13.04,24.1 10.65,26.48 U1.12
  Top 0.305: R1.2 13.33,22.09 Q4.1
C1
  Top 0.152: R2.2 16.22,23.15 16.01,23.36 14.21,23.36 12.17,25.4 U1.13
  Top 0.305: R2.2 16.51,22.09 Q1.1
C2
  Top 0.152: R3.2 19.39,22.86 18.59,23.67 14.34,23.67 12.67,25.33 U1.14
  Top 0.305: R3.2 19.68,22.09 Q2.1
C3
  Top 0.152: U1.15 13.12,28.39 13.12,25.31 14.46,23.97 18.73,23.97 19.26,23.44 21.78,23.44 22.57,22.65 R4.2
  Top 0.305: R4.2 22.86,22.09 Q3.1
C4  (via drill 0.35)
  Top 0.152: v13.73,26.43 13.73,28.38 U1.16 | R5.2 9.44,17.53 12.05,17.53 v13.57,19.05
  Top 0.305: Q5.1 9.07,17.31 R5.2
  Bottom 0.152: v13.73,26.43 13.18,25.88 13.18,19.45 v13.57,19.05
C5  (via drill 0.35)
  Top 0.152: U1.17 14.17,27.25 14.34,27.08 14.34,26.01 v13.81,25.48 | v14.63,19.28 14.63,18.6 13.26,17.22 11.03,17.22 10.48,16.67 10.48,15.53 R6.2
  Top 0.305: Q6.1 9.07,14.13 R6.2
  Bottom 0.152: v13.81,25.48 13.81,20.1 v14.63,19.28
C6
  Top 0.152: R7.2 25.74,22.78 25.4,23.12 22.53,23.12 21.23,24.42 21.23,31.07 20.36,31.95 U1.29
  Top 0.305: R7.2 26.03,22.09 Q7.1
C7
  Top 0.152: U1.30 20.33,32.45 21.54,31.25 21.54,24.54 22.65,23.43 28.19,23.43 28.92,22.7 R8.2
  Top 0.305: R8.2 29.21,22.09 Q8.1
C8
  Top 0.152: U1.31 20.47,32.95 21.84,31.57 21.84,24.67 22.78,23.73 30.74,23.73 R9.2
  Top 0.305: R9.2 32.38,22.09 Q9.1
C9  (via drill 0.35)
  Top 0.152: R10.2 13.99,17.22 15.64,17.22 16.49,18.08 v16.49,18.8 | U1.39 16.67,32.44 15.45,31.22 15.45,30.85 14.45,29.84 v12.86,29.84
  Top 0.305: R10.2 13.49,16.14 Q10.1
  Bottom 0.152: v16.49,18.8 16.49,22.56 14.58,24.48 14.58,26.45 12.86,28.16 v12.86,29.84
C10  (via drill 0.35)
  Top 0.152: R11.2 16.38,17.25 v17.14,18.02 | U1.40 16.17,32.44 15.13,31.4 15.13,31.02 14.59,30.48 v13.81,30.48
  Top 0.305: R11.2 16.67,16.14 Q11.1
  Bottom 0.152: v13.81,30.48 13.81,27.64 14.88,26.57 14.88,25.12 17.14,22.86 v17.14,18.02
C11  (via drill 0.35)
  Top 0.152: R12.2 19.63,16.51 19.63,17.93 v19.64,17.94 | v14.45,31.27 14.75,31.58 14.78,31.58 15.67,32.47 U1.41
  Top 0.305: R12.2 19.84,16.14 Q12.1
  Bottom 0.152: v19.64,17.94 19.64,21 15.19,25.45 15.19,26.7 14.45,27.44 v14.45,31.27
C12  (via drill 0.35)
  Top 0.152: R14.2 25.9,17.33 v25.96,17.38 | U1.25 19.19,29.37 20,28.56 20,26.35 18.91,25.25 18.5,25.25 18.49,25.24 v18.06,25.24
  Top 0.305: R14.2 26.19,16.14 Q14.1
  Bottom 0.152: v25.96,17.38 25.96,18.34 24.84,19.45 23.1,19.45 23.01,19.54 23.01,19.57 21.64,20.94 21.6,20.94 18.06,24.48 v18.06,25.24
C13  (via drill 0.35)
  Top 0.152: U1.26 20.03,30.45 20.31,30.17 20.31,26.23 19.03,24.95 19.02,24.95 18.75,24.69 v18.75,24.65 | v22.7,17.38 22.73,17.36 R13.2
  Top 0.305: R13.2 23.02,16.14 Q13.1
  Bottom 0.152: v18.75,24.65 18.75,25.41 18.31,25.85 17.81,25.85 17.45,25.49 17.45,24.99 17.46,24.98 17.46,24.13 22.7,18.89 v22.7,17.38
C14  (via drill 0.35)
  Top 0.152: U1.27 20.24,30.95 20.62,30.57 20.62,26.11 19.53,25.01 v19.53,24.05 | v29.21,18.73 29.21,16.57 R15.2
  Top 0.305: R15.2 29.37,16.14 Q15.1
  Bottom 0.152: v19.53,24.05 19.57,24.05 23.69,19.94 24.69,19.94 24.7,19.92 28.02,19.92 v29.21,18.73
C15  (via drill 0.35)
  Top 0.152: v32.23,17.38 32.17,17.33 R16.2 | U1.28 20.25,31.45 20.93,30.78 20.93,25.3 v20.56,24.92
  Top 0.305: Q16.1 32.54,15.67 32.48,15.73 32.48,16.12 R16.2
  Bottom 0.152: v32.23,17.38 32.23,17.73 29.24,20.72 24.77,20.72 v20.56,24.92
CHARG  (via drill 0.35)
  Top 0.152: U2.1 17.63,8.89 v17.31,9.21 | v14.53,32.18 14.22,31.88 14.2,31.88 12.77,30.45 U1.11
  Bottom 0.152: v17.31,9.21 21.4,13.29 25.97,13.29 30.69,18.02 30.69,18.76 29.21,20.24 24.38,20.24 18.47,26.15 17.68,26.15 16.72,25.19 16.18,25.19 15.49,25.88 15.49,26.93 15.05,27.36 15.05,31.66 v14.53,32.18
CLK  (via drill 0.35)
  Top 0.152: U4.3 34.08,26.48 v34.01,26.56 33.37,26.56 32.03,27.9 32.03,29.58 33.79,31.34 33.79,32.84 34.48,33.53 34.48,34.76 34.78,35.06 U3.3 | U5.3 34.9,17.91 v34.69,17.7 | U1.22 v16.67,29.76 v16.67,29.77
  Bottom 0.152: v34.01,26.56 34.08,26.48 34.08,25.05 35.29,23.84 35.29,18.31 v34.69,17.7 26.79,25.6 22.27,25.6 18.46,29.41 17.02,29.41 v16.67,29.77
DATA_B  (via drill 0.35)
  Top 0.152: U5.2 34.73,18.56 v34.69,18.61 | U1.20 15.67,29.71 16.34,30.37 17.33,30.37 v17.62,30.08
  Bottom 0.152: v34.69,18.61 27.39,25.9 22.4,25.9 18.23,30.07 17.63,30.07 v17.62,30.08
DATA_G  (via drill 0.35)
  Top 0.152: U1.19 15.17,29.64 16.53,31 v17.86,31 | v23.65,26.59 v28.97,26.59 | v32.7,28.34 32.7,27.8 33.33,27.16 35.63,27.16 U4.2
  Bottom 0.152: v32.7,28.34 30.72,28.34 v28.97,26.59 | v17.86,31 22.27,26.59 v23.65,26.59
DATA_R  (via drill 0.35)
  Top 0.152: U3.2 35.1,35.71 34.85,35.96 34.85,40.01 32.86,41.99 v28.26,41.99 | v19.37,36.51 18.49,36.51 17.11,35.12 17.11,32.44 15.76,31.1 15.76,30.65 14.67,29.57 U1.18
  Bottom 0.152: v19.37,36.51 18.41,36.51 17.7,37.23 17.7,38.02 18.02,38.34 21.45,38.34 21.58,38.21 27.09,38.21 28.26,39.37 v28.26,41.99
G0  (via drill 0.35)
  Top 0.152: U4.5 34.25,25.18 31.73,27.71 31.73,29.71 33.48,31.46 33.48,32.97 34.18,33.66 34.18,39.96 33.18,40.96 28.26,40.96 27.54,41.67 v27.54,45.24
  Bottom 0.152: P1.1 25,46.57 26.32,45.24 v27.54,45.24
G1  (via drill 0.35)
  Top 0.152: v30.56,40.24 33.18,40.24 33.87,39.55 33.87,33.78 33.18,33.09 33.18,31.59 31.42,29.83 31.42,27.59 34.47,24.53 U4.6
  Bottom 0.152: v30.56,40.24 30.59,40.28 P1.4
G2  (via drill 0.35)
  Top 0.152: U4.7 34.69,23.88 31.11,27.46 31.11,29.96 32.87,31.72 32.87,33.22 33.57,33.91 33.57,38.73 v32.77,39.52
  Bottom 0.152: v32.77,39.52 35.88,42.63 P1.7
G3  (via drill 0.35)
  Top 0.152: U4.8 34.91,23.23 30.81,27.33 30.81,30.09 32.07,31.34 v32.07,33.34
  Bottom 0.152: P1.10 40.26,43.29 38.22,41.26 37.79,41.26 32.07,35.53 v32.07,33.34
G4  (via drill 0.35)
  Top 0.152: U4.9 36.2,22.58 36.5,22.89 36.5,28.74 37.97,30.21 37.97,30.69 38.97,31.69 38.97,36.84 39.85,37.72 v39.85,39.21
  Bottom 0.152: v39.85,39.21 39.89,39.17 P1.13
G5  (via drill 0.35)
  Top 0.152: U4.10 36.51,21.93 36.8,22.23 36.8,28.61 38.28,30.09 38.28,30.56 39.85,32.13 v39.85,35.24
  Bottom 0.152: P1.16 46.69,34.26 45.7,35.24 v39.85,35.24
G6  (via drill 0.35)
  Top 0.152: U4.11 36.46,21.28 37.11,21.94 37.11,28.06 v38.02,28.97
  Bottom 0.152: P1.19 47.21,30.33 39.38,30.33 v38.02,28.97
G7  (via drill 0.35)
  Top 0.152: U4.12 36.12,20.63 v37.07,19.68
  Bottom 0.152: P1.22 48.01,23.22 44.5,19.71 40.22,19.71 38.29,21.64 37.69,21.64 37.07,21.02 v37.07,19.68
G8  (via drill 0.35)
  Top 0.152: v45.48,18.97 45.48,20.32 44.53,21.27 42.94,21.27 42.3,20.63 U4.13
  Bottom 0.152: v45.48,18.97 46.57,18.97 P1.25
G9  (via drill 0.35)
  Top 0.152: U4.14 42.52,21.28 42.82,21.58 44.66,21.58 46.09,20.14 46.09,16.4 v44.45,14.76
  Bottom 0.152: P1.28 45.5,13.72 v44.45,14.76
G10  (via drill 0.35)
  Top 0.152: U4.15 44.9,21.93 46.39,20.44 46.39,15.76 43.77,13.13 43.77,12.64 42.09,10.95 v41.51,10.95
  Bottom 0.152: v41.51,10.95 41.51,8.65 P1.31
G11  (via drill 0.35)
  Top 0.152: v38.02,7.14 38.71,7.14 44.08,12.51 44.08,13.01 46.7,15.63 46.7,20.57 44.68,22.58 U4.16
  Bottom 0.152: v38.02,7.14 37.6,6.73 P1.34
G12  (via drill 0.35)
  Top 0.152: U4.17 44.46,23.23 47,20.69 47,15.5 44.38,12.88 44.38,12.39 38.45,6.46 37.4,6.46 35.95,5 v32.54,5
  Bottom 0.152: v32.54,5 32.54,2.33 P1.37
G13  (via drill 0.35)
  Top 0.152: U4.18 44.24,23.88 47.31,20.82 47.31,15.38 44.69,12.76 44.69,12.26 38.54,6.11 37.49,6.11 33.92,2.54 v27.54,2.54
  Bottom 0.152: v27.54,2.54 27.54,1.74 P1.40
G14  (via drill 0.35)
  Top 0.152: v22.23,2.38 22.77,1.83 27.69,1.83 27.87,2.01 33.82,2.01 37.6,5.79 38.65,5.79 44.99,12.13 44.99,12.61 47.61,15.23 47.61,20.95 44.02,24.53 U4.19
  Bottom 0.152: v22.23,2.38 21.35,1.51 P1.43
GND  (via drill 0.35)
  Top 0.152: IC8.9 24.52,29.71 C18.2 v24.02,28.34 | IC8.11 25.52,30.09 25.8,29.81 26.07,29.81 26.67,29.21 C19.2 v26.71,28.34 | IC8.18 27.21,33.63 C20.2 v28.73,32.98 | IC8.1 v22.07,33.63 | C21.2 v24.16,36.43 | U5.1 35.08,19.21 v34.69,19.61
  Top 0.305: U1.35 20.57,34.95 C11.2 | U1.23 17.17,26.84 C8.2 v16.27,26.75 | U4.1 v33.98,27.78 v33.97,27.78 | U3.1 35.56,36.45 v35.56,37.31 | U1.8 11.71,31.95 12.35,32.59 v12.38,32.59 | U1.47 12.67,35.94 12.49,35.76 12.49,35.12 v13.05,34.56
  Top 0.508: v45.48,18.02 R19.1 44.26,18.27 C3.2 44.26,20.28 v44.21,20.32 | v45.56,26.59 R18.1 44.26,26.84 C2.2 44.26,33.78 44.53,34.05 44.51,34.08 R17.1 44.26,35.41 C1.2 44.26,37.02 v43.97,37.31 | C11.2 v20.88,33.66 | C10.2 v6.35,30.88 | C9.2 C7.2 5.27,38.53 5.87,39.13 v6.92,39.13 | Y1.2 v4.76,34.37 | C12.2 12.56,40.21 R47.1 12.54,40.35 v12.54,41.2 | T1.E 18.27,37.71 v18.35,37.62 | X3.1 13.31,10.18 R53.1 15.53,10.18 C14.2 16.59,10.24 R49.1 19.29,9.31 19.29,7.94 | C15.2 24.48,8.62 24.4,8.62 23.35,9.68 C13.2 | IC7.2 26.59,8.73 25.64,7.78 C15.2 | 19.29,7.94 19.29,6.59 20,5.87 21.53,5.87 21.95,6.3 22.49,6.3 22.78,6.59 25.48,6.59 | U2.2 19.29,7.94 | C15.2 25.48,7.62 25.48,6.59 | USB1.12 8.25,21.31 USB1.D | USB1.A 8.25,28.69 USB1.1 | C16.2 30.48,6.59 v29.13,6.59 25.48,6.59 | USB1.B USB1.C
  Bottom 0.508: v26.71,28.34 26.71,32.94 | 26.71,32.94 26.71,33.88 25.89,34.7 24.21,34.7 | v28.73,32.98 26.76,32.98 26.71,32.94 | v24.02,28.34 v26.71,28.34 | 24.21,34.7 23.14,34.7 v22.07,33.63 20.9,33.63 v20.88,33.66 | 24.21,34.7 24.21,36.39 v24.16,36.43 24.16,37.62 | 12.54,41.91 v12.54,41.2 12.39,41.05 12.39,34.53 | 12.54,41.91 12.54,45.4 P1.74 | 24.21,44.05 X2.1 16.4,42.83 15.48,41.91 12.54,41.91 | v18.35,37.62 24.16,37.62 | v44.21,20.32 44.21,25.24 v45.56,26.59 | USB1.B 4.68,29.32 | 4.68,29.32 6.35,29.32 | 6.35,29.32 USB1.A 9.12,29.32 v12.38,32.59 12.38,33.5 12.39,33.51 12.39,34.53 | USB1.C USB1.D | v45.48,18.02 40.56,18.02 38.92,16.38 38.92,15.52 30.2,6.8 29.34,6.8 v29.13,6.59 | v34.69,19.61 33.14,21.15 33.14,22.62 | v6.35,30.88 6.35,29.32 | v6.92,39.13 6.92,36.53 v4.76,34.37 4.76,29.4 4.68,29.32 | 12.39,34.53 13.02,34.53 v13.05,34.56 13.54,34.56 14.39,33.71 15.93,33.71 17.07,34.85 18.34,34.85 18.86,34.32 18.86,32.43 18.26,31.83 16.59,31.83 15.72,30.96 15.72,28.97 16.27,28.42 v16.27,26.75 | 24.16,37.62 27.7,37.62 29.05,38.97 29.05,42.47 27.46,44.05 24.21,44.05 | SV1.1 24.21,44.05 | 33.14,22.62 31.83,22.62 26.71,27.74 v26.71,28.34 | 33.14,22.62 33.14,26.95 v33.97,27.78 33.97,31.99 33.66,32.3 33.66,35.41 v35.56,37.31 36.35,38.1 38.97,38.1 39.72,37.35 43.93,37.35 v43.97,37.31
  other vias: 21.59,43.18 20.32,43.18 21.59,44.45 22.86,44.45 22.86,43.18 22.86,41.91 22.86,40.64 24.13,40.64 24.13,41.91 24.13,43.18 24.13,44.45 25.4,44.45 25.4,43.18 25.4,41.91 25.4,40.64 25.4,39.37 26.67,39.37 26.67,40.64 27.94,38.1 29.21,38.1 29.21,35.56 27.94,35.56 26.67,35.56 27.94,34.29 29.21,34.29 29.21,31.75 3.81,33.02 3.81,31.75 5.08,31.75 5.08,30.48 3.81,30.48 3.81,27.94 2.54,27.94 2.54,26.67 3.81,26.67 11.43,24.13 10.16,24.13 10.16,22.86 8.89,10.16 17.78,3.81 30.48,11.43 45.72,24.13 46.99,24.13 45.72,25.4 44.45,25.4 22.86,48.26 21.59,48.26 17.78,45.72 17.78,44.45 17.78,43.18 16.51,45.72 15.24,45.72 12.7,43.18
  pour Bottom (isolate 0.152): 0,25 arc-90 25,50 arc-90 50,25 arc-90 25,0 arc-90
  pour Top (isolate 0.152): 0,25 arc-90 25,50 arc-90 50,25 arc-90 25,0 arc-90
LOAD  (via drill 0.35)
  Top 0.152: v34.69,25.88 35.62,25.88 U4.4 | U3.4 35.26,34.41 34.94,34.08 34.94,33.11 v34.61,32.78 | U1.21 16.17,27.62 15.67,27.12 15.67,27 15.66,27 15.66,26.1 15.97,25.8 v16.43,25.8 | v36.75,17.86 36.15,17.26 U5.4
  Bottom 0.152: v34.61,32.78 34.66,32.73 34.66,25.9 v34.69,25.88 35.6,24.96 35.6,17.86 | 35.6,17.86 35.6,17.46 35.23,17.09 34.44,17.09 26.24,25.29 22.15,25.29 20.05,27.38 18.02,27.38 v16.43,25.8 | v36.75,17.86 35.6,17.86
N$1
  Top 0.305: U3.23 42.26,35.71 R17.2
N$2
  Top 0.305: U4.23 42.26,27.13 R18.2
N$3
  Top 0.305: U5.23 42.26,18.56 R19.2
N$4
  Top 0.305: T1.C 23.42,39.69 26.83,36.27 BZ1.2
N$5
  Top 0.305: R20.1 17.9,40.27 T1.B
N$49
  Top 0.305: U1.1 10.65,36.17 9.94,36.88 9.94,38.1 8.45,39.59 8.45,41.23 11.27,44.05 X2.2
N$50  (via drill 0.35)
  Top 0.152: Q16.3 31.48,13.1 v30.64,13.1
  Bottom 0.152: v30.64,13.1 29.45,13.1 28.02,11.67 25.1,11.67 20.29,6.86 15.58,6.86 15.57,6.88 15.07,6.88 14.56,6.38 14.56,5.44 15.93,4.08 P1.46
N$51
  Top 0.508: U2.5 20.51,9.79 R49.2
N$52
  Top 0.152: IC8.10 25.02,29.71 C19.1
N$53
  Top 0.152: C21.1 25.52,35.33 IC8.20
N$54  (via drill 0.35)
  Top 0.152: Q15.3 27.62,12.41 v27.62,12.3
  Bottom 0.152: P1.47 14.22,6.46 14.94,7.18 15.7,7.18 15.71,7.17 20.17,7.17 25.3,12.3 v27.62,12.3
N$55
  Top 0.508: X3.2 12.3,6.11 12.96,5.46 16.03,5.46 | U2.3 16.83,6.99 C14.1 16.11,7.7 16.11,5.54 16.03,5.46 | S1.2 25.78,5.09 25.24,5.64 22.23,5.64 21.51,4.92 18.34,4.92 17.8,5.46 16.03,5.46
N$56  (via drill 0.35)
  Top 0.152: Q14.3 24.26,12.22 v23.81,12.22
  Bottom 0.152: P1.48 12.58,5.25 14.82,7.49 15.82,7.49 15.84,7.47 19.06,7.47 v23.81,12.22
N$57  (via drill 0.35)
  Top 0.152: Q13.3 v22.07,12.3
  Bottom 0.152: P1.49 12.54,5.64 14.69,7.79 15.95,7.79 15.96,7.78 17.54,7.78 v22.07,12.3
N$58  (via drill 0.35)
  Top 0.152: Q12.3 v18.89,12.22
  Bottom 0.152: P1.50 9.53,8.02 11.76,10.25 16.92,10.25 v18.89,12.22
N$59  (via drill 0.35)
  Top 0.152: Q11.3 v15.72,12.22
  Bottom 0.152: v15.72,12.22 14.05,10.56 10.63,10.56 P1.51
N$60  (via drill 0.35)
  Top 0.152: Q10.3 v12.54,12.22
  Bottom 0.152: P1.52 9.63,12.22 v12.54,12.22
N$61  (via drill 0.35)
  Top 0.152: Q9.3 30.69,18.41 v30.08,18.41
  Bottom 0.152: P1.53 8.37,13.6 25.27,13.6 v30.08,18.41
N$62  (via drill 0.35)
  Top 0.152: Q8.3 v28.26,18.18
  Bottom 0.152: P1.54 6.06,13.9 23.98,13.9 v28.26,18.18
N$63  (via drill 0.35)
  Top 0.152: Q7.3 v25.08,18.18
  Bottom 0.152: v25.08,18.18 21.11,14.21 3.81,14.21 P1.55
N$64  (via drill 0.35)
  Top 0.152: Q6.3 5.24,15.08 v5.16,15.16
  Bottom 0.152: P1.56 4.48,15.84 v5.16,15.16
N$65  (via drill 0.35)
  Top 0.152: Q5.3 5.24,18.26 v5.16,18.34
  Bottom 0.152: v5.16,18.34 3.02,18.34 P1.57
N$66  (via drill 0.35)
  Top 0.152: Q3.3 v21.91,18.18
  Bottom 0.152: P1.58 5.2,19.41 7.5,17.11 20.84,17.11 v21.91,18.18
N$67  (via drill 0.35)
  Top 0.152: Q2.3 v18.73,18.18
  Bottom 0.152: P1.59 1.51,21.25 2.91,22.65 7.94,22.65 10.52,20.07 10.52,18.83 11.94,17.41 17.97,17.41 v18.73,18.18
N$68  (via drill 0.35)
  Top 0.152: Q1.3 v15.56,18.1
  Bottom 0.152: P1.60 7.9,23.12 10.82,20.2 10.82,18.96 11.68,18.1 v15.56,18.1
N$69  (via drill 0.35)
  Top 0.152: Q4.3 11.48,19.16 v11.43,19.21
  Bottom 0.152: P1.61 6.45,25 11.43,20.02 v11.43,19.21
OE
  Top 0.152: U5.21 41,17.26 40.77,17.49 40.77,21.65 40.76,21.66 40.76,25.85 | 40.76,25.85 40.76,28.14 41.12,28.5 41.91,28.5 42.39,28.97 42.39,34.13 42.11,34.41 U3.21 40.84,34.41 40.64,34.61 40.64,39.75 36.42,43.97 29.99,43.97 26.89,47.07 15,47.07 13.34,45.4 11.91,45.4 8.06,41.56 8.06,39.29 9.48,37.87 9.48,35.21 9.74,34.95 U1.2 | U4.21 40.78,25.83 40.76,25.85
OSC32_IN
  Top 0.152: U1.3 9.76,34.45 9.18,35.04 9.18,37.21 Y2.1 6.59,37.89 C7.1
OSC32_OUT
  Top 0.152: U1.4 9.47,33.95 9.25,34.17 9.07,34.35 8.49,34.92 Y2.2 8.49,36.51 C9.1
OSC_IN
  Top 0.152: Y1.1 6.99,35.32 8.85,33.45 U1.5
OSC_OUT
  Top 0.152: U1.6 8.16,32.95 7.7,33.42 Y1.3
R0  (via drill 0.35)
  Top 0.152: U3.5 36.61,33.76 36.91,34.05 36.91,39.45 33.73,42.62 30.48,42.62 v28.81,44.29
  Bottom 0.152: P1.3 28.81,48.65 v28.81,44.29
R1  (via drill 0.35)
  Top 0.152: U3.6 36.4,33.11 37.21,33.93 37.21,40.26 v34.13,43.34
  Bottom 0.152: v34.13,43.34 34.13,47.16 P1.6
R2  (via drill 0.35)
  Top 0.152: v37.54,41.99 37.52,41.96 37.52,33.62 36.35,32.46 U3.7
  Bottom 0.152: P1.9 37.54,42.91 v37.54,41.99
R3  (via drill 0.35)
  Top 0.152: U3.8 36.27,31.81 37.82,33.36 37.82,39.17 v38.26,39.61
  Bottom 0.152: v38.26,39.61 39.29,40.64 P1.12
R4  (via drill 0.35)
  Top 0.152: v38.5,37.31 38.5,33.29 36.36,31.16 U3.9
  Bottom 0.152: v38.5,37.31 39.84,35.97 P1.15
R5  (via drill 0.35)
  Top 0.152: U3.10 36.22,30.51 37.54,31.83 v38.26,31.83
  Bottom 0.152: v38.26,31.83 39,31.08 47.93,31.08 P1.18
R6  (via drill 0.35)
  Top 0.152: U3.11 36.6,29.86 v36.75,30
  Bottom 0.152: v36.75,30 36.75,27.4 37.77,26.38 39.08,26.38 42.42,29.73 44.37,29.73 P1.21
R7  (via drill 0.35)
  Top 0.152: U3.12 35.56,29.11 v35.56,28.57 | v46.67,25.48 48.35,23.8 P1.24
  Bottom 0.152: v35.56,28.57 35.56,27.7 37.19,26.08 39.25,26.08 42.6,29.42 44.16,29.42 46.67,26.91 v46.67,25.48
  other vias: 48.35,19.5
R8  (via drill 0.35)
  Top 0.152: U3.13 40.72,29.21 40.46,28.94 40.46,21.54 40.47,21.53 40.47,16.26 v39.93,15.72
  Bottom 0.152: v39.93,15.72 44.91,15.72 P1.27
R9  (via drill 0.35)
  Top 0.152: U3.14 40.43,29.86 40.15,29.58 40.15,21.41 40.16,21.4 40.16,16.81 39.16,15.81 v39.16,14.32
  Bottom 0.152: v39.16,14.32 40.53,14.32 41.94,12.91 41.94,12.45 43.29,11.09 P1.30
R10  (via drill 0.35)
  Top 0.152: U3.15 40.56,30.51 39.85,29.79 39.85,21.28 39.86,21.27 39.86,16.94 38.56,15.64 38.56,13.59 v38.89,13.26
  Bottom 0.152: v38.89,13.26 39.25,12.9 39.25,5.78 P1.33
R11  (via drill 0.35)
  Top 0.152: U3.16 40.72,31.16 39.54,29.98 39.54,21.16 39.55,21.15 39.55,17.06 38.25,15.76 38.25,12.5 v38.6,12.14
  Bottom 0.152: P1.36 34.26,6.36 38.6,10.7 v38.6,12.14
R12  (via drill 0.35)
  Top 0.152: U3.17 40.82,31.81 39.24,30.23 39.24,21.03 39.25,21.02 39.25,17.19 37.95,15.89 37.95,10.9 v37.52,10.48
  Bottom 0.152: P1.39 28.84,1.8 29.77,2.73 30.02,2.73 31.94,4.65 31.94,5.25 32.29,5.61 32.65,5.61 v37.52,10.48
R13  (via drill 0.35)
  Top 0.152: U3.18 41.04,32.46 38.93,30.35 38.93,20.91 38.94,20.9 38.94,17.31 37.64,16.02 37.64,12.08 v36.2,10.64
  Bottom 0.152: v36.2,10.64 29.13,3.57 25.8,3.57 23.39,1.17 P1.42
R14  (via drill 0.35)
  Top 0.152: U3.19 41,33.11 40.3,32.41 40.3,32.15 38.63,30.48 38.63,20.78 38.64,20.77 38.64,17.44 37.34,16.14 37.34,12.3 36.36,11.32 36.02,11.32 v35.05,10.35
  Bottom 0.152: P1.45 19.57,4.13 28.83,4.13 v35.05,10.35
RESET
  Top 0.305: U1.7 8.78,32.45 R46.1
SCL  (via drill 0.35)
  Top 0.152: R51.1 15.17,38.88 U1.42 15.17,34.95 v14.71,34.49 13.87,33.65 12.55,33.65 11.63,34.56 11.63,35.7 11.19,36.14 11.19,36.2 10.48,36.91 10.48,38.1 9.13,39.45 v9.13,40.4 | v23.26,36.27 23.34,36.19 23.34,35.08 23.56,34.86 23.73,34.86 24.03,34.57 24.03,34.3 IC8.23
  Bottom 0.152: v14.71,34.49 14.32,34.49 13.81,35 13.81,35.88 14.21,36.27 16.13,36.27 16.5,35.91 20.47,35.91 21.35,36.79 22.21,36.79 22.72,36.27 v23.26,36.27 | v9.13,40.4 8.08,41.45 P1.71
SDA  (via drill 0.35)
  Top 0.152: R50.1 14.67,38.25 U1.43 14.67,35.79 v14.45,35.56 13.81,34.92 13.81,34.37 13.39,33.95 12.67,33.95 12.11,34.52 12.11,35.75 10.78,37.08 10.78,38.23 9.76,39.24 v9.76,41.12 | IC8.24 23.1,34.28 22.7,34.69 v22.7,35.4
  Bottom 0.152: v22.7,35.4 22.7,35.86 22.08,36.48 21.48,36.48 20.55,35.56 v14.45,35.56 | v9.76,41.12 9.76,42.92 P1.72
SWCLK
  Top 0.152: SV1.3 19.2,45.89 19.2,37.29 18.87,36.97 U1.37
SWDIO
  Top 0.152: SV1.2 19.54,43.83 19.54,37.2 19.97,36.76 19.97,36.26 19.62,35.91 18.42,35.91 17.94,35.42 17.94,34.7 18.18,34.45 U1.34
USB_DM  (via drill 0.35)
  Top 0.152: v17.77,33.09 v17.78,33.09 18.14,33.45 U1.32 | USB1.7 7.48,24.75 7.3,24.92 7.3,25.56 7.54,25.8 8.2,25.8 USB1.5 9.32,25.75 v9.84,26.27
  Bottom 0.152: v9.84,26.27 9.84,28.87 14.06,33.09 16.89,33.09 v17.77,33.09
USB_DP  (via drill 0.35)
  Top 0.152: U1.33 17.82,33.95 v17.78,34 | USB1.6 9.29,25.25 | 9.29,25.25 9.29,24.45 9.09,24.25 USB1.8 | 9.29,25.25 v9.83,25.25 v9.84,25.24
  Bottom 0.152: v9.84,25.24 10.48,25.88 10.48,29.08 14.19,32.79 16.76,32.79 16.96,32.59 17.16,32.39 18.02,32.39 18.38,32.74 18.38,33.4 v17.78,34
V_SENS
  Top 0.152: 14.32,8.18 9.13,8.18 3.89,13.41 3.89,18.97 5.08,20.16 5.08,28.89 6.43,30.24 9.13,30.24 9.84,30.95 U1.10
  Top 0.508: R52.1 14.32,8.18 14.32,8.84 R53.2
VBUS
  Top 0.305: USB1.11 7.56,22.6 7.38,22.78 6.43,22.78 | 6.43,26.27 7.62,27.46 8.18,27.46 USB1.2
  Top 0.508: U2.4 20.8,6.99 21.59,7.78 | C13.1 21.59,7.78 | 21.59,7.78 21.59,10.87 21.03,11.43 6.83,11.43 4.37,13.88 4.37,18.77 5.64,20.03 5.64,21.99 6.43,22.78 6.43,26.27

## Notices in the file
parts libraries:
my_Wurth_Quartz Crystals: Copyright: Würth Elektronik
